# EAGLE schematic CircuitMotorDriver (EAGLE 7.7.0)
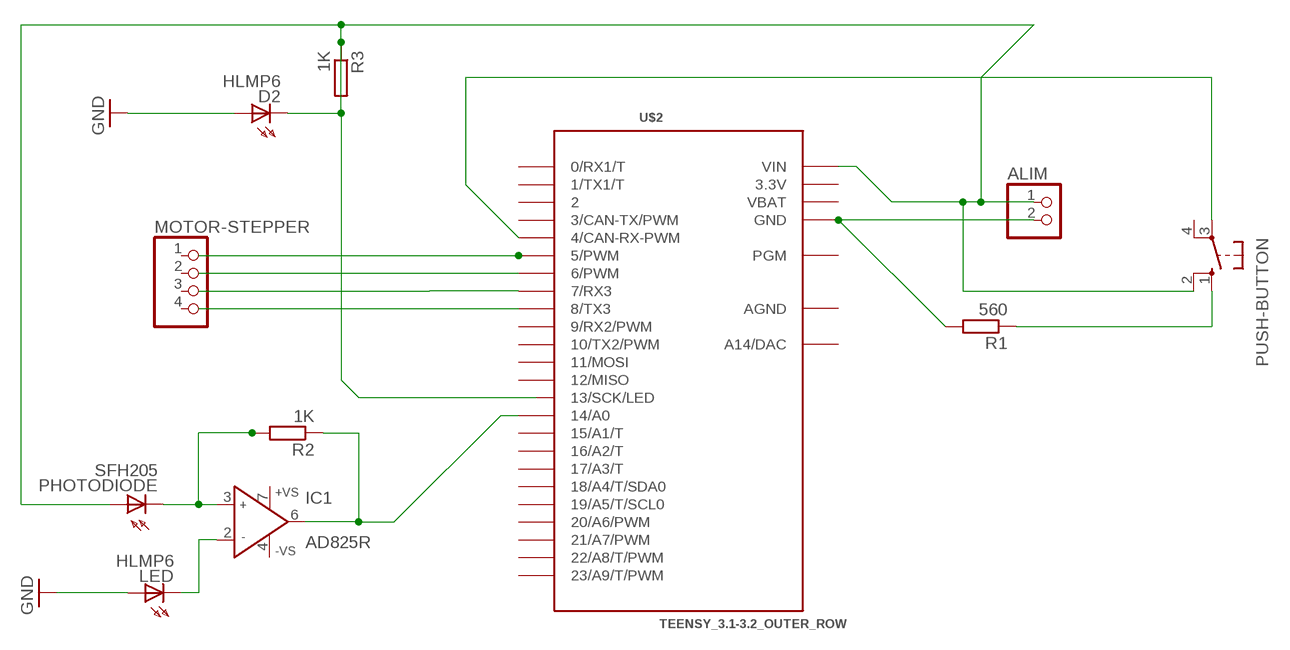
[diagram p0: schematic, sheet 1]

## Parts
ALIM  PINHD-1X2  [1X02]
D2  HLMP6  [HLMP6]
IC1  AD825R  [SO8]
LED  HLMP6  [HLMP6]
MOTOR-STEPPER  PINHD-1X4  [1X04]
PHOTODIODE  SFH205  [SFH205]
PUSH-BUTTON  10-XX  [B3F-10XX]
R1  560  R-EU_0411/12  [0411/12]
R2  1K  R-EU_0411/12  [0411/12]
R3  1K  R-EU_0411/12  [0411/12]
U$2  TEENSY_3.1-3.2_OUTER_ROW  [TEENSY_3.0-3.2&LC_OUTER_ROW]

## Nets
GND: ALIM.1 D2.A D2.K PHOTODIODE.A PUSH-BUTTON.2(S1) R3.1 R3.2 U$2.VIN
MOTOR-STEPPER: U$2.5(5/PWM)
N$2: U$2.6(6/PWM)
N$3: U$2.7(7/RX3)
N$4: U$2.8(8/TX3)
N$5: ALIM.2 R1.2 U$2.GND U$2.GND1(GND)
N$6: IC1.3(IN+) PHOTODIODE.K(C) R2.2
N$7: PUSH-BUTTON.1(S) R1.1
N$8: IC1.6(OUT) R2.1 U$2.14/A0
N$9: PUSH-BUTTON.3(P) U$2.4(4/CAN-RX-PWM)
N$11: IC1.2(IN-) LED.K
N$12: LED.A ; supply symbol labelled GND
Unconnected: IC1.4(-VS) IC1.7(+VS) MOTOR-STEPPER.1 MOTOR-STEPPER.2 MOTOR-STEPPER.3 MOTOR-STEPPER.4 PUSH-BUTTON.4(P1) U$2.0(0/RX1/T) U$2.1(1/TX1/T) U$2.2 U$2.3(3/CAN-TX/PWM) U$2.9(9/RX2/PWM) U$2.10(10/TX2/PWM) U$2.11(11/MOSI) U$2.12(12/MISO) U$2.13(13/SCK/LED) U$2.15/A1(15/A1/T) U$2.16/A2(16/A2/T) U$2.17/A3(17/A3/T) U$2.18/A4(18/A4/T/SDA0) U$2.19/A5(19/A5/T/SCL0) U$2.20/A6(20/A6/PWM) U$2.21/A7(21/A7/PWM) U$2.22/A8(22/A8/T/PWM) U$2.23/A9(23/A9/T/PWM) U$2.PGM U$2.RESET/DAC(A14/DAC)

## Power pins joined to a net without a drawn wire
3.3V: U$2.3.3V U$2.3.3V1(3.3V)
AGND: U$2.AGND
VBAT: U$2.VBAT

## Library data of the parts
ALIM = pinhead:PINHD-1X2: PIN HEADER
D2 LED = display-hp:HLMP6: LED; MF: AGILENT TECHNOLOGIES; MPN: HLMP-6500; OC_FARNELL: 1652490; OC_NEWARK: 40K0088
IC1 = analog-devices:AD825: Low Cost, General-Purpose High Speed JFET Amplifier Source: http://www.analog.com/static/imported-files/data_sheets/AD825.pdf; MF: ALTERA CORPORATION; MPN: AD825ARZ; OC_FARNELL: 9603735; OC_NEWARK: 59K6528
MOTOR-STEPPER = pinhead:PINHD-1X4: PIN HEADER
PHOTODIODE = opto-trans-siemens:SFH205: PHOTO DIODE; OC_FARNELL: unknown; OC_NEWARK: unknown
PUSH-BUTTON = switch-omron:10-XX: OMRON SWITCH; MPN: B3F-1000; OC_FARNELL: 176432; OC_NEWARK: 36M3542
R1-R3 = resistor:R-EU_: RESISTOR, European symbol
U$2 = Teensy_3_and_LC_Series_Boards_v1.4:TEENSY_3.1-3.2_OUTER_ROW: Footprint for Teensy 3.1 or 3.2 board using all pin connections on the outer perimeter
